(* Logix 5000 DataType export EdDSA_MSG; software revision 30.00 *)

TYPE EdDSA_MSG :
STRUCT
   Status : CONNECTION_STATUS;
   Flags : DINT;
   PubDH : STRING;
   Ke : STRING;
   KsID : LINT;
   KsPrimeID : LINT;
   Counter : LINT;
   Sig_R : STRING;
   Sig_S : STRING;
END_STRUCT
END_TYPE
